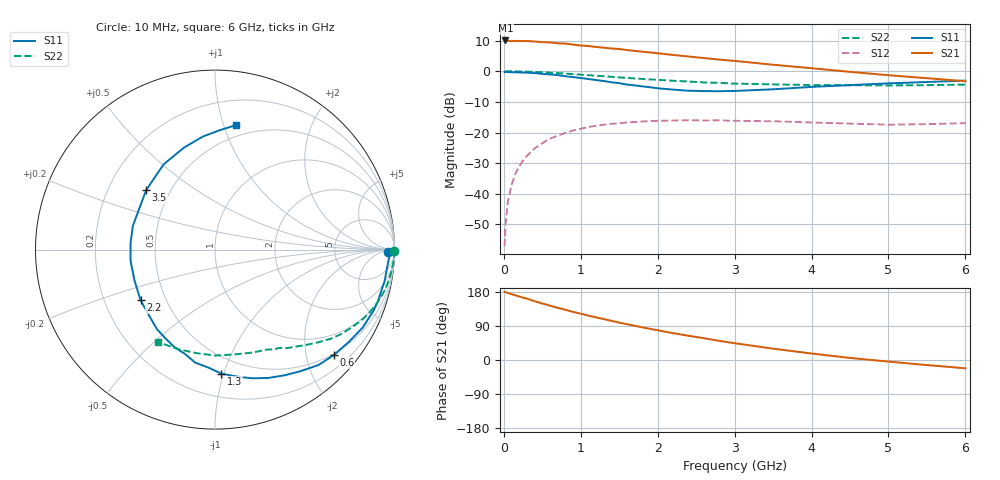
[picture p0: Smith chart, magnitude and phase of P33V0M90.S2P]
! SIEMENS Small Signal Semiconductors
! BFP181
! Si NPN RF Bipolar Junction Transistor in SOT143
! VCE = 3 V  IC = 0.9 mA
! Common Emitter S-Parameters:  March  1996
# GHz  S  MA  R  50
!  f  S11  S21  S12  S22
! GHz  MAG  ANG  MAG  ANG  MAG  ANG  MAG  ANG
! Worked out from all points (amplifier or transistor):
!   36 points, 10 MHz to 6 GHz, reference 50 ohm
!   highest |S21| = 10.0 dB at 20 MHz (marker M1)
!   |S21| within 3 dB of that: start of sweep to 1.565 GHz
!   unconditionally stable (mu >= 1): 3.227 GHz to end of sweep
!   at 250 MHz: K = 0.09, MSG = 19.5 dB, |S12| = -29.2 dB
!   at 1.4 GHz: K = 0.48, MSG = 12.3 dB, |S12| = -17.2 dB
!   at 6 GHz: K = 1.29, MAG = 3.6 dB, |S12| = -16.9 dB
!   S11 on the Smith chart (normalised r, x): 10 MHz: 50, -21; 600 MHz: 0.47, -2.56; 1.3 GHz: 0.37, -0.98; 2.2 GHz: 0.36, -0.27; 3.5 GHz: 0.37, +0.33; 6 GHz: 0.40, +1.10
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0.01  0.9666 -0.8  3.124 179.7  0.0014 82.5  0.9983 -0.3
0.02  0.9748 -1.5  3.174 179.5  0.0029 89.0  0.9979 -0.6
0.05  0.969 -3.3  3.136 177.0  0.0072 90.3  0.9976 -1.7
0.1  0.963 -7.0  3.093 173.9  0.0139 82.9  0.9979 -3.3
0.2  0.9545 -14.0  3.119 167.6  0.0281 80.0  0.9915 -6.5
0.3  0.9466 -21.0  3.108 162.0  0.0416 75.9  0.9836 -9.8
0.4  0.9307 -27.8  3.051 155.2  0.055 71.6  0.9745 -13.0
0.6  0.8853 -41.5  2.953 143.4  0.0793 62.6  0.9476 -18.9
0.8  0.8276 -55.0  2.822 132.5  0.0986 54.3  0.9153 -24.4
1.1  0.7455 -74.1  2.577 117.0  0.1228 43.4  0.8612 -31.6
1.3  0.6917 -87.1  2.419 107.9  0.1342 36.9  0.8276 -35.9
1.5  0.6389 -100.0  2.302 98.7  0.142 31.4  0.7917 -39.7
1.8  0.5653 -119.5  2.084 86.1  0.1511 24.3  0.7486 -44.6
2.2  0.5015 -145.8  1.842 70.8  0.1569 15.9  0.6982 -50.9
2.4  0.4803 -159.1  1.738 64.0  0.1586 12.4  0.6796 -53.9
2.8  0.4718 175.8  1.546 50.5  0.1578 6.8  0.6458 -59.5
3  0.4764 163.9  1.473 44.3  0.1553 4.3  0.6275 -62.6
3.5  0.5069 139.2  1.275 29.9  0.1526 -0.2  0.6101 -70.2
4  0.5545 121.1  1.119 17.1  0.1457 -3.2  0.5941 -79.3
4.5  0.5937 107.0  0.976 5.5  0.1398 -5.3  0.5905 -89.5
5.5  0.6663 87.6  0.77 -13.4  0.1367 -1.3  0.592 -110.7
6  0.7029 80.5  0.687 -21.9  0.1423 -0.2  0.605 -121.7
